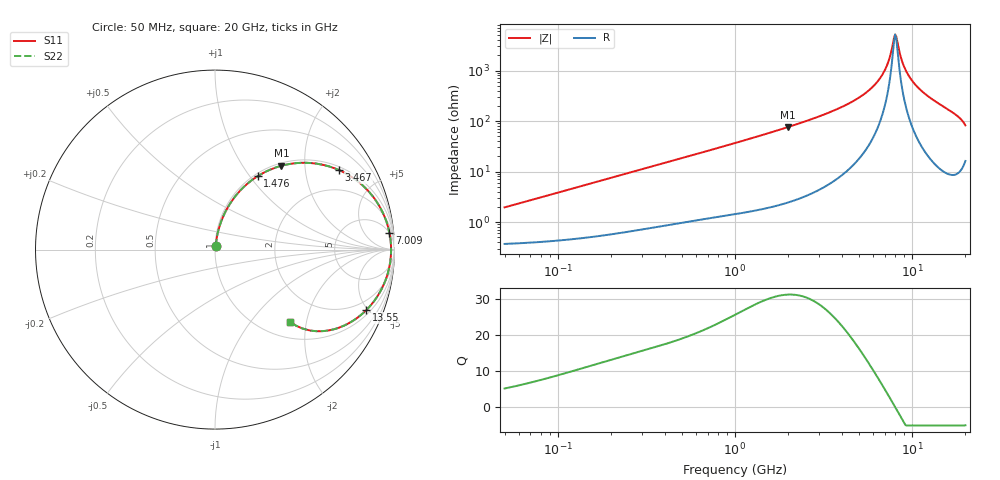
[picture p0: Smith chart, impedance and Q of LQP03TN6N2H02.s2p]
!Murata Part Number: LQP03TN6N2H02
!These Parameters are Measured in Series Mode Connection
!  o--[Z]--o
!Port1  Port2
!  o-------o
!Freq. Start=50[MHz] Stop=20[GHz], 401[Steps]
# Hz S RI R 50
!Freq.(Hz) S11(Real) S11(Imag) S21(Real) S21(Imag) S12(Real) S12(Imag) S22(Real) S22(Imag)
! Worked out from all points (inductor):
!   401 points, 50 MHz to 20 GHz, reference 50 ohm
!   read as one part in series: L = 6.1 nH near 51.52 MHz
!   highest Q = 31.1 at 1.992 GHz (marker M1), where L = 6.07 nH
!   self-resonance near 8.021 GHz
!   S11 on the Smith chart (normalised r, x): 50 MHz: 1.01, +0.04; 1.476 GHz: 1.04, +1.10; 3.467 GHz: 1.12, +3.03; 7.009 GHz: 5, +20; 13.55 GHz: 1.27, -4.88; 20 GHz: 1.32, -1.61
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5e7  0.00405 0.0191  0.996 -0.0191  0.996 -0.0191  0.00405 0.0191
1.364002e8  0.00741 0.051  0.9926 -0.051  0.9926 -0.051  0.00741 0.051
3.721004e8  0.0262 0.133  0.9738 -0.133  0.9738 -0.133  0.0262 0.133
1e9  0.1279 0.3149  0.8721 -0.3149  0.8721 -0.3149  0.1279 0.3149
1.476162e9  0.2386 0.4097  0.7614 -0.4097  0.7614 -0.4097  0.2386 0.4097
1.99176e9  0.3698 0.4669  0.6302 -0.4669  0.6302 -0.4669  0.3698 0.4669
2.728004e9  0.5462 0.4812  0.4538 -0.4812  0.4538 -0.4812  0.5462 0.4812
3.466789e9  0.6903 0.4434  0.3097 -0.4434  0.3097 -0.4434  0.6903 0.4434
4.472136e9  0.8287 0.3521  0.1713 -0.3521  0.1713 -0.3521  0.8287 0.3521
5.433528e9  0.9103 0.2515  0.0897 -0.2515  0.0897 -0.2515  0.9103 0.2515
6.311513e9  0.9534 0.1609  0.0466 -0.1609  0.0466 -0.1609  0.9534 0.1609
7.009217e9  0.972 0.0927  0.028 -0.0927  0.028 -0.0927  0.972 0.0927
7.442007e9  0.9782 0.0526  0.0218 -0.0526  0.0218 -0.0526  0.9782 0.0526
7.901521e9  0.9809 0.0119  0.0191 -0.0119  0.0191 -0.0119  0.9809 0.0119
8.141811e9  0.981 -0.00851  0.019 0.00851  0.019 0.00851  0.981 -0.00851
8.907419e9  0.9761 -0.07  0.0239 0.07  0.0239 0.07  0.9761 -0.07
9.745021e9  0.9631 -0.131  0.0369 0.131  0.0369 0.131  0.9631 -0.131
1.115139e10  0.9283 -0.2198  0.0717 0.2198  0.0717 0.2198  0.9283 -0.2198
1.354865e10  0.8431 -0.3369  0.1569 0.3369  0.1569 0.3369  0.8431 -0.3369
1.696185e10  0.6761 -0.4398  0.3239 0.4398  0.3239 0.4398  0.6761 -0.4398
1.855685e10  0.5647 -0.4545  0.4353 0.4545  0.4353 0.4545  0.5647 -0.4545
2e10  0.4182 -0.4027  0.5818 0.4027  0.5818 0.4027  0.4182 -0.4027
